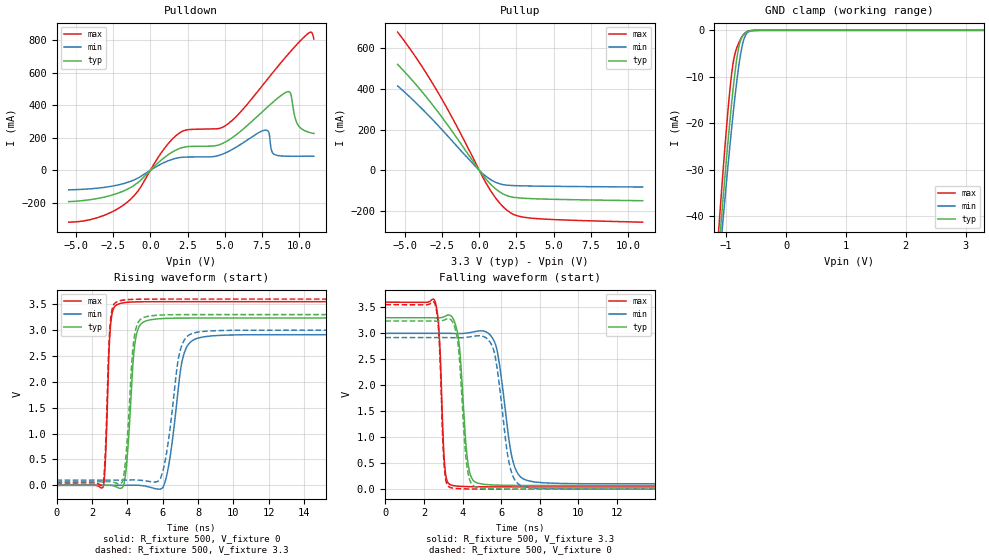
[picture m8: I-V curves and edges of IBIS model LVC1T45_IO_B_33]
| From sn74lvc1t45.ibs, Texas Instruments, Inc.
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[Model]   LVC1T45_IO_B_33
Model_type  I/O
Vinl=0.8
Vinh=2.0
Enable   Active-Low
Vref =   0
Rref =   2000
Cref =   15p
Vmeas =   1.65
| variable   typ   min   max
C_comp   6.86pF   5.92pF   8.14pF
| C_pullup   10.82pF   9.16pF   12.69pF
| C_pulldown   10.11pF   7.31pF   13.23pF
| C_tri-state   6.86pF   5.92pF   8.14pF
[Temperature Range]   40   100   -40
| Ambient temperature   25   85   -40
[Voltage range]   3.3   3   3.6
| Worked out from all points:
|   slope of the pulldown table from 0 to 0.495 V, typ, clamps not added: 11.2 ohm
|   slope of the pullup table from 0 to 0.495 V, typ, clamps not added: 10.6 ohm
|   GND clamp passes 1 mA (typ) near -0.71 V on its own axis
|   rising waveform, R_fixture 500, V_fixture 0: 20-80 % time 360ps typ, 624ps min, 211ps max; typ from 0 V to 3.23 V
|   falling waveform, R_fixture 500, V_fixture 3.3: 20-80 % time 352ps typ, 619ps min, 218ps max; typ from 3.3 V to 0.069 V
|   rising waveform, R_fixture 500, V_fixture 3.3: 20-80 % time 358ps typ, 630ps min, 216ps max; typ from 0.069 V to 3.3 V
|   falling waveform, R_fixture 500, V_fixture 0: 20-80 % time 344ps typ, 584ps min, 213ps max; typ from 3.24 V to 0 V
[GND Clamp]
| LVC1T45_IO_B_33
|   Voltage   I(typ)   I(min)   I(max)
-5.5V     -910.9mA   -836.3mA   -1.031A
-1.12V    -47.12mA   -50.9mA    -42.25mA
-1.09V    -42.34mA   -46.45mA   -36.95mA
-1.06V    -37.63mA   -42.05mA   -31.78mA
-950mV    -21.32mA   -26.62mA   -14.52mA
-910mV    -15.92mA   -21.37mA   -9.573mA
-875mV    -11.59mA   -17mA      -6.417mA
-820mV    -5.939mA   -10.75mA   -3.68mA
-770mV    -2.643mA   -6.035mA   -2.191mA
-710mV    -920.7uA   -2.212mA   -923.3uA
-635mV    -221.2uA   -410.8uA   -171uA
3.3V      10.41pA    35.81nA    8.12pA
[Pulldown]
| LVC1T45_IO_B_33
|   Voltage   I(typ)   I(min)   I(max)
-5.5V     -194.6mA   -121.5mA   -321.3mA
-1.825V   -129.3mA   -83.52mA   -216.3mA
1.7V      123.2mA    72.65mA    211.3mA
5V        171.2mA    104.3mA    271.8mA
7.675V    372mA      246.2mA    537.6mA
7.97V     396.6mA    233.5mA    571.4mA
8.25V     419.5mA    102.9mA    603.3mA
9.215V    483.4mA    85.88mA    709.4mA
9.445V    469.9mA    85.7mA     733.5mA
9.93V     278.8mA    85.68mA    782.4mA
10.77V    230.9mA    85.86mA    851.2mA
11V       225.9mA    85.92mA    808.7mA
[Pullup]
| LVC1T45_IO_B_33
|   Voltage   I(typ)   I(min)   I(max)
-5.5V     521mA      415.5mA    680.3mA
-4.125V   410.3mA    322.3mA    540.3mA
-2.79V    288.4mA    222mA      384.5mA
-1.5V     158.2mA    118.3mA    215mA
195mV     -19.51mA   -13.56mA   -27.85mA
640mV     -58.63mA   -39.42mA   -85.46mA
1.07V     -88.98mA   -57.5mA    -132.8mA
1.49V     -111.1mA   -68.41mA   -170.4mA
1.9V      -125.3mA   -73.08mA   -198.2mA
2.575V    -134.8mA   -75.52mA   -223.8mA
3.665V    -139.5mA   -77.22mA   -236mA
11V       -149.3mA   -81.96mA   -254.9mA
[Ramp]
| LVC1T45_IO_B_33
| variable   typ   min   max
dV/dt_r   1.98/3.73E-10   1.79/6.46E-10   2.16/2.23E-10
dV/dt_f   1.97/3.66E-10   1.77/6.35E-10   2.17/2.33E-10
R_load = 500
[Rising Waveform]
| LVC1T45_IO_B_33
R_fixture =   500
C_fixture =   0
L_fixture =   0
V_fixture =   0
V_fixture_min = 0
V_fixture_max = 0
|   Time   V(typ)   V(min)   V(max)
0s        168.9pV    331.3pV    105.2pV
2.635ns   535.9uV    -2.868uV   -26.37mV
3.05ns    328.1uV    25.36uV    3.071V
3.53ns    -54.06mV   -143.3uV   3.507V
3.92ns    272.3mV    949.2uV    3.534V
4.46ns    2.808V     3.006mV    3.545V
5.03ns    3.175V     -15.41mV   3.548V
6.095ns   3.225V     21.1mV     3.549V
7.925ns   3.233V     2.839V     3.55V
29.99ns   3.234V     2.914V     3.55V
[Falling Waveform]
| LVC1T45_IO_B_33
R_fixture =   500
C_fixture =   0
L_fixture =   0
V_fixture =   3.3
V_fixture_min = 3
V_fixture_max = 3.6
|   Time   V(typ)   V(min)   V(max)
0s        3.3V       3V         3.6V
2.575ns   3.298V     3V         3.617V
3.075ns   3.325V     3V         462.9mV
3.415ns   3.333V     2.999V     78.23mV
4.295ns   465.1mV    3.009V     49.31mV
4.77ns    118.4mV    3.043V     46.61mV
5.725ns   78.71mV    2.768V     44.83mV
6.58ns    72.54mV    585.1mV    44.39mV
7.355ns   70.73mV    166.2mV    44.25mV
29.99ns   69.38mV    100.9mV    44.1mV
[Rising Waveform]
| LVC1T45_IO_B_33
R_fixture =   500
C_fixture =   0
L_fixture =   0
V_fixture =   3.3
V_fixture_min = 3
V_fixture_max = 3.6
|   Time   V(typ)   V(min)   V(max)
0s        69.31mV    100.8mV    44.06mV
2.615ns   69.7mV     100.8mV    24.07mV
3.03ns    70.18mV    100.8mV    3.107V
3.485ns   30.06mV    100.6mV    3.558V
3.87ns    372.7mV    101.5mV    3.584V
4.385ns   2.846V     103.5mV    3.595V
4.945ns   3.247V     90.25mV    3.598V
5.93ns    3.291V     181.5mV    3.6V
7.7ns     3.3V       2.94V      3.6V
29.99ns   3.3V       3V         3.6V
[Falling Waveform]
| LVC1T45_IO_B_33
R_fixture =   500
C_fixture =   0
L_fixture =   0
V_fixture =   0
V_fixture_min = 0
V_fixture_max = 0
|   Time   V(typ)   V(min)   V(max)
0s        3.237V     2.918V     3.551V
2.57ns    3.235V     2.918V     3.567V
3.06ns    3.258V     2.918V     399.8mV
3.37ns    3.272V     2.917V     31mV
4.26ns    360.9mV    2.925V     4.439mV
4.705ns   39.48mV    2.951V     2.252mV
5.615ns   7.22mV     2.675V     712.3uV
6.42ns    2.499mV    493.6mV    318.2uV
7.135ns   1.128mV    52.09mV    185.7uV
29.99ns   70.31uV    137.7uV    35.21uV
